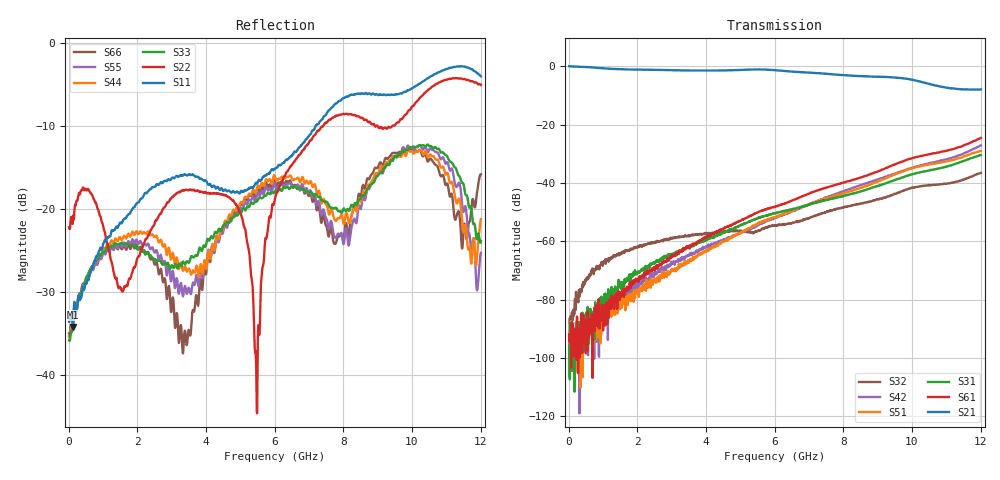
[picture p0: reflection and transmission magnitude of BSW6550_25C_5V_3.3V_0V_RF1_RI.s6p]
! Agilent Technologies	N5230C	MY49001333	A.09.33.09
!	Test time	=	2026-05-06 10:00
!	Product	=	BSW6550
!	Temp	=	25C
!	VDD	=	5
!	Control_High	=	3.3
!	Control_Low	=	0
!	Logic	=	RF1
!	Port1	=	RFC
!	Port2	=	RF1
!	Port3	=	RF2
!	Port4	=	RF3
!	Port5	=	RF4
!	Port6	=	RF5
!	V1	=	3.3 / 0
!	V2	=	3.3 / 0
!	V3	=	3.3 / 0
!S6P File: Measurements: <S11,S12,S13,S14,S15,S16>,
!<S21,S22,S23,S24,S25,S26>,
!<S31,S32,S33,S34,S35,S36>,
!<S41,S42,S43,S44,S45,S46>,
!<S51,S52,S53,S54,S55,S56>,
!<S61,S62,S63,S64,S65,S66>;
# HZ S RI R 50
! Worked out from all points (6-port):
!   1201 points, 10 MHz to 12.01 GHz, reference 50 ohm
!   strongest paths, dB at 10 MHz, 3.01 GHz, 6.01 GHz, 9.01 GHz, 12.01 GHz:
!     S21: 0.1, -1.3, -1.3, -3.6, -7.9
!     S61: -91.9, -64.9, -48.1, -36.1, -24.6
!     S31: -100.0, -64.4, -50.4, -41.0, -30.4
!     S51: -94.4, -69.5, -51.7, -39.5, -29.0
!     S42: -106.2, -67.7, -52.0, -38.8, -27.1
!     S32: -103.8, -58.8, -54.7, -45.7, -36.5
!   lowest |S11| = -34.2 dB at 120 MHz (marker M1), VSWR 1.04, Z = 51.9 - j0.609 ohm
!   |S11| at or under -10 dB: start of sweep to 7.194 GHz
